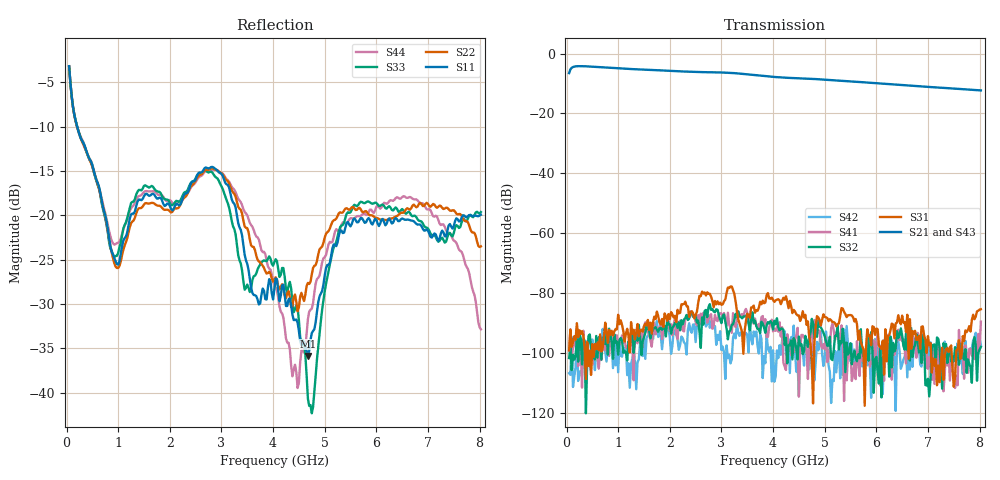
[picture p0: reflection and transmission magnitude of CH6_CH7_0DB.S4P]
!Agilent Technologies,E5071C,MY46316741,A.11.02
!Date: Mon Jun 01 10:32:44 2026
!Data & Calibration Information:
!1:CH6 INPUT 2:CH6 OUTPUT 3:CH7 INPUT 4:CH7 OUTPUT
!Freq	S11:SOLT4(ON)	S12:SOLT4(ON)	S13:SOLT4(ON)	S14:SOLT4(ON)
!	S21:SOLT4(ON)	S22:SOLT4(ON)	S23:SOLT4(ON)	S24:SOLT4(ON)
!	S31:SOLT4(ON)	S32:SOLT4(ON)	S33:SOLT4(ON)	S34:SOLT4(ON)
!	S41:SOLT4(ON)	S42:SOLT4(ON)	S43:SOLT4(ON)	S44:SOLT4(ON)
!PortZ  Port1:50+j0  Port2:50+j0  Port3:50+j0  Port4:50+j0
!Above PortZ is port z conversion or system Z0 setting when saving the data.
!When reading, reference impedance value at option line is always used.
# Hz S dB R 50
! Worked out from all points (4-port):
!   320 points, 50 MHz to 8.025 GHz, reference 50 ohm
!   strongest paths, dB at 50 MHz, 2.05 GHz, 4.05 GHz, 6.05 GHz, 8.025 GHz:
!     S21: -6.5, -5.8, -7.8, -10.0, -12.3
!     S43: -6.5, -5.8, -7.9, -10.1, -12.4
!     S31: -99.1, -87.1, -82.4, -97.6, -85.4
!     S32: -101.7, -91.6, -90.4, -110.2, -98.0
!     S41: -99.1, -94.1, -92.6, -97.0, -89.5
!     S42: -106.8, -97.6, -108.0, -105.4, -97.4
!   lowest |S11| = -35.9 dB at 4.675 GHz (marker M1), VSWR 1.03, Z = 49 - j1.27 ohm
!   |S11| at or under -10 dB: 206.8 MHz to end of sweep
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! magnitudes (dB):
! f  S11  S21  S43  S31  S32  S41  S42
! 50 MHz  -3.2  -6.5  -6.5  -99.1  -101.7  -99.1  -106.8
! 975 MHz  -25.5  -4.9  -4.9  -92.1  -96.2  -94.1  -96.5
! 2.8 GHz  -14.5  -6.2  -6.2  -81.2  -85.6  -87.0  -89.3
! 4.475 GHz  -32.1  -8.2  -8.3  -87.5  -102.2  -91.6  -103.5
! 4.675 GHz  -35.9  -8.4  -8.5  -89.5  -98.0  -108.7  -104.1
! 5.575 GHz  -20.3  -9.4  -9.4  -89.5  -99.3  -103.3  -98.8
! 8.025 GHz  -19.9  -12.3  -12.4  -85.4  -98.0  -89.5  -97.4
